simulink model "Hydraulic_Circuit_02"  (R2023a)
settings: Solver=VariableStepAuto  StartTime=0.0  StopTime=10.0  RelTol=1e-3
libraries: fl_lib x11

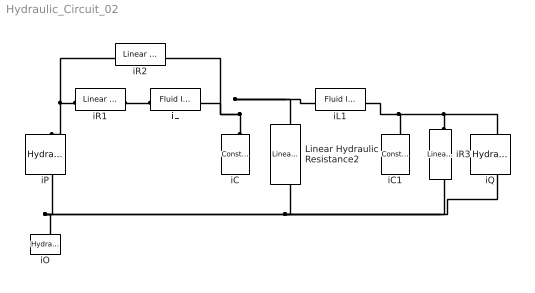
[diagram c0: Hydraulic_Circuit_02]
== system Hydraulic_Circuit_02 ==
  Linear Hydraulic Resistance2 : fl_lib/Hydraulic/Hydraulic Elements/Linear Hydraulic Resistance  resistance=10e9 Pa*s/m^3  q_specify=off  q_priority=None  q=1e-3 m^3/s  q_nominal_specify=off  q_nominal_unit=m^3/s  q_nominal_value=1  p_specify=off  p_priority=None  p=0 Pa  p_nominal_specify=off  p_nominal_unit=Pa  p_nominal_value=1
  iC : fl_lib/Hydraulic/Hydraulic Elements/Constant Volume Hydraulic Chamber  ch_sp=foundation.enum.chamberGeometry.volume  wall_type=foundation.enum.chamber_spec.rigid  ch_volume=1e-4 m^3  d_in=1e-2 m  length=1 m  pr_r_coef=1.2e-12 m/Pa  time_const=0.01 s  k_sh=1.4  pressure_specify=off  pressure_priority=High  pressure=0 Pa  pressure_nominal_specify=off  pressure_nominal_unit=Pa  pressure_nominal_value=1  diameter_incr_specify=off  diameter_incr_priority=High  diameter_incr=0 m  diameter_incr_nominal_specify=off  diameter_incr_nominal_unit=m  diameter_incr_nominal_value=1  flow_rate_specify=off  flow_rate_priority=None  flow_rate=1e-3 m^3/s  flow_rate_nominal_specify=off  flow_rate_nominal_unit=m^3/s  flow_rate_nominal_value=1
  iC1 : fl_lib/Hydraulic/Hydraulic Elements/Constant Volume Hydraulic Chamber  ch_sp=foundation.enum.chamberGeometry.volume  wall_type=foundation.enum.chamber_spec.rigid  ch_volume=1e-4 m^3  d_in=1e-2 m  length=1 m  pr_r_coef=1.2e-12 m/Pa  time_const=0.01 s  k_sh=1.4  pressure_specify=off  pressure_priority=High  pressure=0 Pa  pressure_nominal_specify=off  pressure_nominal_unit=Pa  pressure_nominal_value=1  diameter_incr_specify=off  diameter_incr_priority=High  diameter_incr=0 m  diameter_incr_nominal_specify=off  diameter_incr_nominal_unit=m  diameter_incr_nominal_value=1  flow_rate_specify=off  flow_rate_priority=None  flow_rate=1e-3 m^3/s  flow_rate_nominal_specify=off  flow_rate_nominal_unit=m^3/s  flow_rate_nominal_value=1
  iL : fl_lib/Hydraulic/Hydraulic Elements/Fluid Inertia  area=0.8e-4 m^2  length=1 m  q_specify=off  q_priority=High  q=1e-3 m^3/s  q_nominal_specify=off  q_nominal_unit=m^3/s  q_nominal_value=1  p_specify=off  p_priority=None  p=0 Pa  p_nominal_specify=off  p_nominal_unit=Pa  p_nominal_value=1
  iL1 : fl_lib/Hydraulic/Hydraulic Elements/Fluid Inertia  area=0.8e-4 m^2  length=1 m  q_specify=off  q_priority=High  q=1e-3 m^3/s  q_nominal_specify=off  q_nominal_unit=m^3/s  q_nominal_value=1  p_specify=off  p_priority=None  p=0 Pa  p_nominal_specify=off  p_nominal_unit=Pa  p_nominal_value=1
  iO : fl_lib/Hydraulic/Hydraulic Elements/Hydraulic Reference
  iP : fl_lib/Hydraulic/Hydraulic Sources/Hydraulic Constant Pressure Source  commanded_pressure=10e5 Pa
  iQ : fl_lib/Hydraulic/Hydraulic Sources/Hydraulic Constant Flow Rate Source  commanded_flow_rate=0.001 m^3/s
  iR1 : fl_lib/Hydraulic/Hydraulic Elements/Linear Hydraulic Resistance  resistance=10e9 Pa*s/m^3  q_specify=off  q_priority=None  q=1e-3 m^3/s  q_nominal_specify=off  q_nominal_unit=m^3/s  q_nominal_value=1  p_specify=off  p_priority=None  p=0 Pa  p_nominal_specify=off  p_nominal_unit=Pa  p_nominal_value=1
  iR2 : fl_lib/Hydraulic/Hydraulic Elements/Linear Hydraulic Resistance  resistance=10e9 Pa*s/m^3  q_specify=off  q_priority=None  q=1e-3 m^3/s  q_nominal_specify=off  q_nominal_unit=m^3/s  q_nominal_value=1  p_specify=off  p_priority=None  p=0 Pa  p_nominal_specify=off  p_nominal_unit=Pa  p_nominal_value=1
  iR3 : fl_lib/Hydraulic/Hydraulic Elements/Linear Hydraulic Resistance  resistance=10e9 Pa*s/m^3  q_specify=off  q_priority=None  q=1e-3 m^3/s  q_nominal_specify=off  q_nominal_unit=m^3/s  q_nominal_value=1  p_specify=off  p_priority=None  p=0 Pa  p_nominal_specify=off  p_nominal_unit=Pa  p_nominal_value=1
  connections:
  iQ/RConn1 -- iR3/RConn1 -- Linear Hydraulic Resistance2/RConn1 -- iP/RConn1 -- iO/LConn1
  iR1/LConn1 -- iP/LConn1 -- iR2/LConn1
  iR1/RConn1 -- iL/LConn1
  iC/LConn1 -- iL1/LConn1 -- Linear Hydraulic Resistance2/LConn1 -- iR2/RConn1 -- iL/RConn1
  iR3/LConn1 -- iQ/LConn1 -- iL1/RConn1 -- iC1/LConn1
